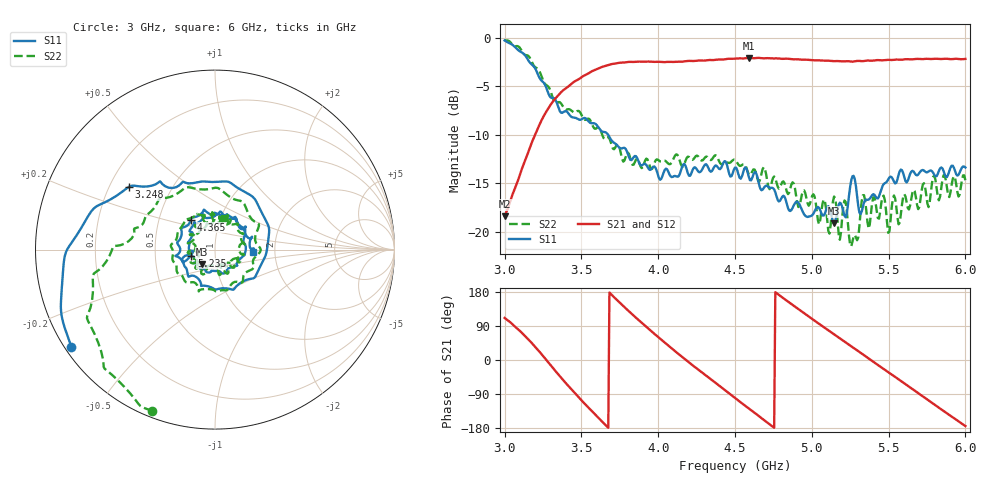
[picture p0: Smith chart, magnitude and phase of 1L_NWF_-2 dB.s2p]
!  26/11/2025  13:31:57
! Ref Plane: 0.000 mm
# MHZ S MA R  50
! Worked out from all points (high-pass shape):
!   401 points, 3 GHz to 6 GHz, reference 50 ohm
!   highest |S21| = -2.09 dB at 4.59 GHz (marker M1); lowest = -18.4 dB at 3 GHz (marker M2)
!   |S21| within 3 dB of the highest: 3.411 GHz to end of sweep
!   lowest |S11| = -19.2 dB at 5.145 GHz (marker M3), VSWR 1.25, Z = 42.6 - j7.02 ohm
!   |S11| at or under -10 dB: 3.673 GHz to end of sweep
!   |S22| runs from -21.5 to -0.3 dB; largest |S21 - S12| = 0.025
!   S11 on the Smith chart (normalised r, x): 3 GHz: 0.02, -0.31; 3.248 GHz: 0.28, +0.30; 4.365 GHz: 0.72, +0.25; 5.235 GHz: 0.76, -0.05; 6 GHz: 1.54, -0.04
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3000  0.9667 -145.8  0.1198 111.0  0.1195 111.8  0.9646 -111.3
3142.5  0.7918 176.3  0.2426 59.4  0.2412 60.5  0.8118 -150.5
3247.5  0.5933 143.8  0.3842 11.8  0.3829 12.5  0.609 -173.8
3360  0.4172 124.7  0.5154 -43.0  0.5141 -42.4  0.4642 165.3
3502.5  0.3797 85.7  0.6267 -107.3  0.6246 -106.5  0.3965 133.4
3622.5  0.3343 40.0  0.7003 -157.5  0.6977 -156.8  0.3364 84.8
3720  0.2844 -5.9  0.7352 162.8  0.732 163.4  0.2706 35.1
3862.5  0.2399 -67.5  0.7515 108.9  0.7489 109.5  0.2378 -25.3
4005  0.1885 -118.5  0.7506 58.9  0.75 59.1  0.2321 -77.2
4185  0.2098 -172.5  0.7567 -1.5  0.7547 0.1  0.2392 -129.4
4365  0.2157 129.0  0.767 -57.7  0.7653 -56.9  0.2453 176.5
4500  0.2137 82.4  0.7784 -100.1  0.7761 -99.3  0.2344 134.1
4590  0.1911 48.3  0.7865 -127.9  0.7812 -127.5  0.1969 104.9
4785  0.1429 -29.4  0.7803 171.9  0.7734 172.8  0.1664 38.7
5002.5  0.1212 -100.0  0.7643 108.3  0.7561 108.8  0.1528 -27.7
5145  0.11 -132.2  0.7562 67.5  0.7484 68.0  0.1515 -62.8
5235  0.1363 -165.9  0.7558 42.1  0.748 42.5  0.1111 -72.5
5370  0.1461 167.1  0.7619 4.0  0.7538 5.0  0.1035 -123.1
5505  0.1899 126.8  0.7675 -34.2  0.7603 -32.7  0.0997 -169.8
5625  0.1827 92.4  0.7742 -68.2  0.7671 -66.5  0.1322 156.7
5745  0.202 62.7  0.7776 -102.3  0.7709 -100.7  0.1549 129.4
6000  0.214 -3.5  0.7764 -174.3  0.7686 -173.4  0.1831 73.9
